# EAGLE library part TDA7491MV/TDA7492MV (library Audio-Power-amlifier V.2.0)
The TDA7491MV is a 25 W mono BTL class-D audio amplifierwith single power supply designed for LCD TVs and monitors. The TDA7492MV is a 50 W mono BTL class-D audio amplifier with single power supply designed for home systems and docking stations.
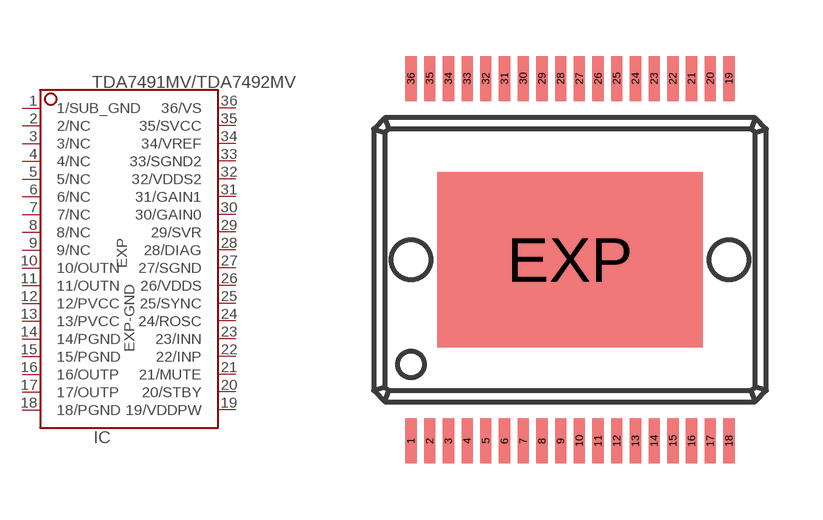
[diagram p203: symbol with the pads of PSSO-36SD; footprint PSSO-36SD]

Designator prefix IC

## TDA7491MV/TDA7492MV  [PSSO-36SD]
1  1/SUB_GND  pwr
2  2/NC  nc
3  3/NC  nc
4  4/NC  nc
5  5/NC  nc
6  6/NC  nc
7  7/NC  nc
8  8/NC  nc
9  9/NC  nc
10  10/OUTN  out
11  11/OUTN  out
12  12/PVCC  pwr
13  13/PVCC  pwr
14  14/PGND  pwr
15  15/PGND  pwr
16  16/OUTP  out
17  17/OUTP  out
18  18/PGND  pwr
19  19/VDDPW  out
20  20/STBY  in
21  21/MUTE  in
22  22/INP  in
23  23/INN  in
24  24/ROSC  out
25  25/SYNC
26  26/VDDS  out
27  27/SGND  pwr
28  28/DIAG  out
29  29/SVR  out
30  30/GAIN0  in
31  31/GAIN1  in
32  32/VDDS2  in
33  33/SGND2  in
34  34/VREF  out
35  35/SVCC  pwr
36  36/VS  out
EXP  EXP-GND  out

## Footprint PSSO-36SD (pad centres in mm)
PowerSSO-36 slug down package
smd 0.3 x 1.2: 1 -4.25,-4.85; 2 -3.75,-4.85; 3 -3.25,-4.85; 4 -2.75,-4.85; 5 -2.25,-4.85; 6 -1.75,-4.85; 7 -1.25,-4.85; 8 -0.75,-4.85; 9 -0.25,-4.85; 10 0.25,-4.85; 11 0.75,-4.85; 12 1.25,-4.85; 13 1.75,-4.85; 14 2.25,-4.85; 15 2.75,-4.85; 16 3.25,-4.85; 17 3.75,-4.85; 18 4.25,-4.85; 19 4.25,4.85; 20 3.75,4.85; 21 3.25,4.85; 22 2.75,4.85; 23 2.25,4.85; 24 1.75,4.85; 25 1.25,4.85; 26 0.75,4.85; 27 0.25,4.85; 28 -0.25,4.85; 29 -0.75,4.85; 30 -1.25,4.85; 31 -1.75,4.85; 32 -2.25,4.85; 33 -2.75,4.85; 34 -3.25,4.85; 35 -3.75,4.85; 36 -4.25,4.85
smd 7.1 x 4.7: EXP 0,0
